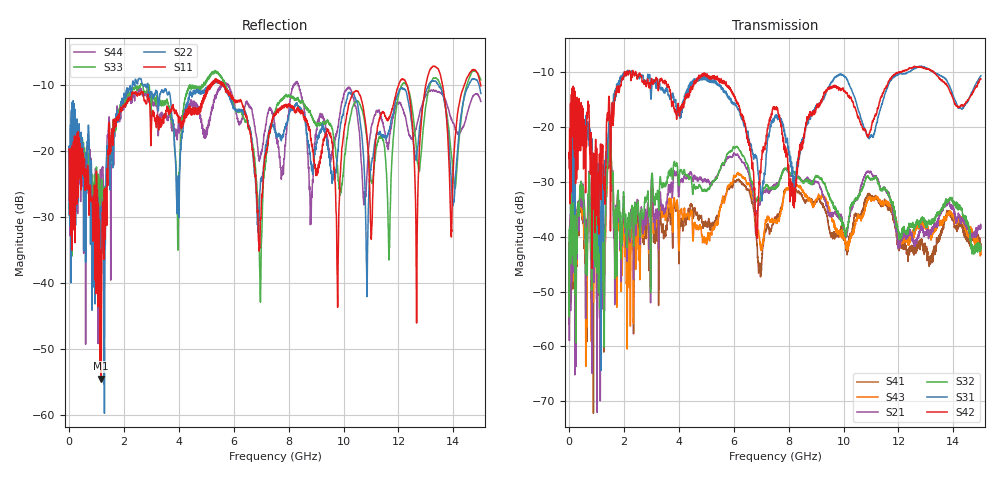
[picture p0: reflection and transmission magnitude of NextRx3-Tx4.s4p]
! FILE: N:\QM 2007\Prüfprotokolle\Highspeed\Konfektionierte Ltg\L45593-D106\D30\8216\0002\Next  Platine 2\NextRx3-Tx4.s4p
# MHz S DB R 50.00
! FREQ  S11  S12  S13  S14
!  S21  S22  S23  S24
!  S31  S32  S33  S34
!  S41  S42  S43  S44
!  DB  ANG  DB  ANG  DB  ANG  DB  ANG
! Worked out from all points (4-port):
!   2999 points, 10 MHz to 15 GHz, reference 50 ohm
!   strongest paths, dB at 10 MHz, 3.755 GHz, 7.505 GHz, 11.26 GHz, 15 GHz:
!     S42: -25.6, -15.8, -16.9, -16.7, -11.3
!     S31: -25.7, -14.8, -18.2, -18.2, -10.7
!     S32: -38.7, -29.1, -31.1, -30.1, -41.9
!     S21: -41.1, -32.0, -30.6, -29.8, -38.4
!     S43: -51.4, -35.7, -37.0, -33.0, -43.2
!     S41: -49.1, -36.7, -36.7, -33.3, -41.9
!   lowest |S11| = -54.4 dB at 1.18 GHz (marker M1), VSWR 1.00, Z = 50.2 + j0.0857 ohm
!   |S11| at or under -10 dB: start of sweep to 5.144 GHz; 5.656 GHz to 12.01 GHz (6.351 GHz wide, 71.9 % of centre); 13.6 GHz to 14.4 GHz (799.7 MHz wide, 5.71 % of centre)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
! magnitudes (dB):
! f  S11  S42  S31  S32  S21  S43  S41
! 10 MHz  -19.7  -25.6  -25.7  -38.7  -41.1  -51.4  -49.1
! 1.18 GHz  -54.4  -28.7  -36.7  -40.2  -37.8  -38.1  -36.1
! 1.48 GHz  -16.6  -15.8  -18.3  -18.9  -19.8  -19.3  -20.2
! 2.135 GHz  -12.8  -9.9  -10.2  -38.1  -39.6  -44.1  -44.1
! 5.675 GHz  -10.5  -12.1  -13.5  -26.3  -26.6  -33.3  -32.9
! 6.84 GHz  -26.5  -38.6  -25.6  -33.2  -35.8  -38.7  -40.7
! 15 GHz  -10.2  -11.3  -10.7  -41.9  -38.4  -43.2  -41.9
